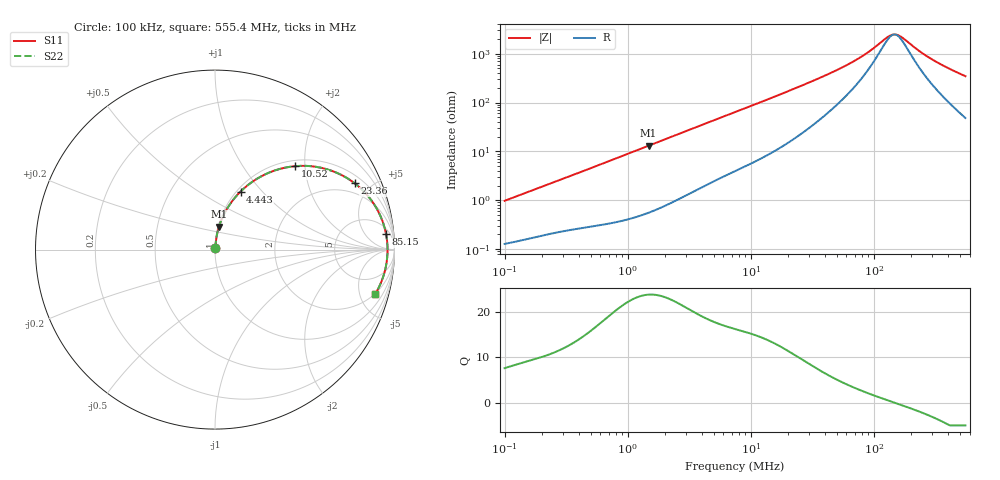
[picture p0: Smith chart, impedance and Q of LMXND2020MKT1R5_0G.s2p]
! LMXND2020MKT1R5_0G  S-PARAMETER MODEL  ( General Type )
! Model Generated by TAIYO YUDEN Corporation (http://www.ty-top.com)
! Version 1.0
! TAIYO YUDEN Control No. 191023NI43SB-FBB
! Copyright(c) 2019 TAIYO YUDEN CO.,LTD. All Rights Reserved.
! Product Description (link to TY-COMPAS)
! https://ds.yuden.co.jp/TYCOMPAS/or/detail?pn=LMXND2020MKT1R5N0G&u=M
! Products Name : Inductors
! Characteristics :
!  Inductance : 1.5 uH , SRF(min) : -Hz , DC Resistance(max) : 0.108 Ohm
!  Rated Current : Saturation :1650 mA , Temp Rise : 1500 mA
!  Case Size : 2.0 x 2.0 / 0.079 x 0.079 [mm/inch] , Thickness : 1.2 / 0.047 [mm/inch]
!  (Conditions: Temperature = 25 degC , DC Bias Current/Voltage = 0A / 0V)
! External Node Assignments :
!  1  o---GGG---o  2
! GND o---------o GND
! Frequency Range : 0.1MHz  -  555.443392MHz  [ 402 STEP ]
# MHz S RI R 50
! Freq[MHz].  S11 Real  S11 Imag  S21 Real  S21 Imag  S12 Real  S12 Imag  S22 Real  S22 Imag
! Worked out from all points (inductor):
!   401 points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, 100 kHz to 555.4 MHz, reference 50 ohm
!   read as one part in series: L = 1.52 uH near 104.4 kHz
!   highest Q = 23.7 at 1.48 MHz (marker M1), where L = 1.41 uH
!   self-resonance near 147.4 MHz
!   S11 on the Smith chart (normalised r, x): 100 kHz: 1.00, +0.02; 4.443 MHz: 1.04, +0.77; 10.52 MHz: 1.12, +1.78; 23.36 MHz: 1.39, +3.97; 85.15 MHz: 9, +18; 555.4 MHz: 1.96, -6.87
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0.1  0.00136 0.00961  0.9986 -0.00961  0.9986 -0.00961  0.00136 0.00961
0.423865  0.00414 0.0381  0.9959 -0.0381  0.9959 -0.0381  0.00414 0.0381
0.826869  0.00894 0.0729  0.9911 -0.0729  0.9911 -0.0729  0.00894 0.0729
1.479789  0.0221 0.1275  0.9779 -0.1275  0.9779 -0.1275  0.0221 0.1275
1.796612  0.0308 0.1529  0.9692 -0.1529  0.9692 -0.1529  0.0308 0.1529
2.949654  0.0727 0.2368  0.9273 -0.2368  0.9273 -0.2368  0.0727 0.2368
4.442644  0.1425 0.3233  0.8575 -0.3233  0.8575 -0.3233  0.1425 0.3233
5.879526  0.2171 0.3839  0.7829 -0.3839  0.7829 -0.3839  0.2171 0.3839
7.615203  0.308 0.4316  0.692 -0.4316  0.692 -0.4316  0.308 0.4316
10.52217  0.4467 0.4649  0.5533 -0.4649  0.5533 -0.4649  0.4467 0.4649
15.17933  0.6141 0.4503  0.3859 -0.4503  0.3859 -0.4503  0.6141 0.4503
23.36064  0.7773 0.3703  0.2227 -0.3703  0.2227 -0.3703  0.7773 0.3703
31.58981  0.8544 0.2962  0.1456 -0.2962  0.1456 -0.2962  0.8544 0.2962
55.32847  0.9302 0.1665  0.0698 -0.1665  0.0698 -0.1665  0.9302 0.1665
85.14921  0.9531 0.0861  0.0469 -0.0861  0.0469 -0.0861  0.9531 0.0861
133.898  0.9611 0.0145  0.0389 -0.0145  0.0389 -0.0145  0.9611 0.0145
145.9556  0.9613 0.00152  0.0387 -0.00152  0.0387 -0.00152  0.9613 0.00152
162.5656  0.9611 -0.0147  0.0389 0.0147  0.0389 0.0147  0.9611 -0.0147
234.5178  0.956 -0.0721  0.044 0.0721  0.044 0.0721  0.956 -0.0721
290.9322  0.9489 -0.1091  0.0511 0.1091  0.0511 0.1091  0.9489 -0.1091
401.9905  0.9297 -0.1719  0.0703 0.1719  0.0703 0.1719  0.9297 -0.1719
555.4434  0.8941 -0.2454  0.1059 0.2454  0.1059 0.2454  0.8941 -0.2454
